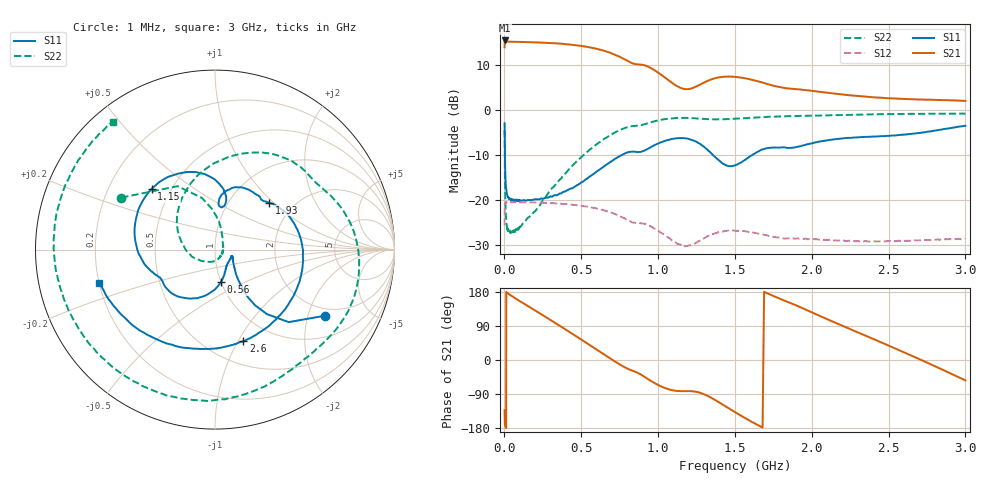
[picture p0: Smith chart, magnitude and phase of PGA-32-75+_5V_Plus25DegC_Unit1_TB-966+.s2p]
!Mini-Circuits Laboratory
!S-Parameters
!Model: PGA-32-75+
!Run / Lot / Date Code: Q18610 / CP621-001-03-01EV / 1724
!Fixture: TB-966+_ED17052601
!Network Analyzer: PNA-X N5244A - 423 4 ports;  Serial number: 74314
!Date: 7/21/2017 at 2:34:57 PM
!S/N: Unit# 1
!Tested with:
# Hz  S  dB  R  50
!Frequency  S11 dB  S11 Deg  S21 dB  S21 Deg  S12 dB  S12 Deg  S22 dB  S22 Deg
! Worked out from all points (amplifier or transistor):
!   399 points, 1 MHz to 3 GHz, reference 50 ohm
!   highest |S21| = 15.4 dB at 2.5 MHz (marker M1)
!   |S21| within 3 dB of that: start of sweep to 708.3 MHz
!   unconditionally stable (mu >= 1): start of sweep to end of sweep
!   at 58 MHz: K = 1.18, MAG = 15.2 dB, |S12| = -20.4 dB
!   at 1.01 GHz: K = 1.58, MAG = 13.1 dB, |S12| = -27.1 dB
!   at 3 GHz: K = 1.54, MAG = 10.9 dB, |S12| = -28.5 dB
!   S11 on the Smith chart (normalised r, x): 1 MHz: 1.71, -2.56; 560 MHz: 1.00, -0.38; 1.15 GHz: 0.39, +0.35; 1.93 GHz: 1.51, +0.94; 2.6 GHz: 0.73, -1.05; 3 GHz: 0.20, -0.13
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1000000  -2.94 -31.2  13.91 -132.4  -25.61 87.2  -4.48 151.0
1500000  -4.79 -44.5  15.20 -149.9  -22.67 63.0  -7.74 120.4
2500000  -8.37 -54.3  15.43 -164.5  -21.24 37.2  -12.81 94.5
8000000  -16.25 -44.4  15.19 -177.8  -20.56 9.4  -22.64 55.4
3.8e7  -19.77 -21.4  15.16 171.4  -20.43 -5.4  -27.07 -7.3
1.4e8  -20.12 -32.3  15.07 145.5  -20.49 -28.0  -24.45 -83.7
2.4e8  -19.61 -45.5  14.96 120.5  -20.53 -49.3  -20.59 -136.3
3.8e8  -18.19 -59.9  14.69 85.2  -20.84 -79.2  -14.60 169.9
5.1e8  -15.92 -73.3  14.17 51.4  -21.27 -107.4  -10.15 130.3
5.6e8  -14.65 -79.8  13.88 38.1  -21.58 -118.6  -8.67 115.6
6.6e8  -12.23 -97.1  13.02 11.5  -22.41 -140.9  -6.19 88.1
7.7e8  -9.87 -123.5  11.47 -16.4  -23.84 -164.1  -4.14 59.3
1.01e9  -7.27 -179.9  8.07 -67.8  -27.06 154.9  -2.23 9.2
1.15e9  -6.21 136.2  4.86 -82.2  -29.86 146.5  -1.74 -17.6
1.38e9  -10.71 77.7  7.13 -107.7  -27.30 129.3  -2.07 -50.4
1.51e9  -12.15 85.0  7.32 -140.0  -26.80 102.5  -1.90 -65.4
1.65e9  -9.24 76.3  6.38 -172.0  -27.43 75.0  -1.63 -82.5
1.93e9  -8.00 41.0  4.54 138.5  -28.57 34.6  -1.29 -118.9
2.01e9  -7.30 32.0  4.22 123.9  -28.62 23.2  -1.24 -129.0
2.51e9  -5.69 -53.3  2.60 36.4  -29.05 -50.5  -0.90 172.3
2.6e9  -5.44 -72.9  2.46 20.4  -28.97 -65.3  -0.87 163.3
3e9  -3.48 -164.1  2.02 -53.8  -28.50 -129.9  -0.82 128.4
